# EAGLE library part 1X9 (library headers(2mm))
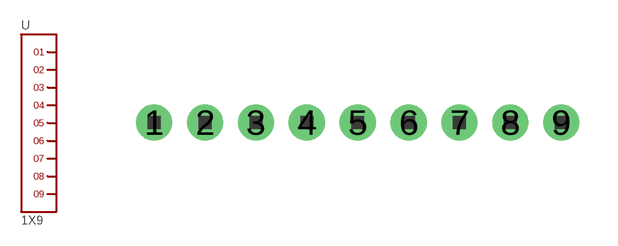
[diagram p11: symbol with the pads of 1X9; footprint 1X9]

Designator prefix -

## 1X9  [1X9]
1  1
2  2
3  3
4  4
5  5
6  6
7  7
8  8
9  9

## Footprint 1X9 (pad centres in mm)
drill 0.8 pad 1.422: 1 -8,0; 2 -6,0; 3 -4,0; 4 -2,0; 5 0,0; 6 2,0; 7 4,0; 8 6,0; 9 8,0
